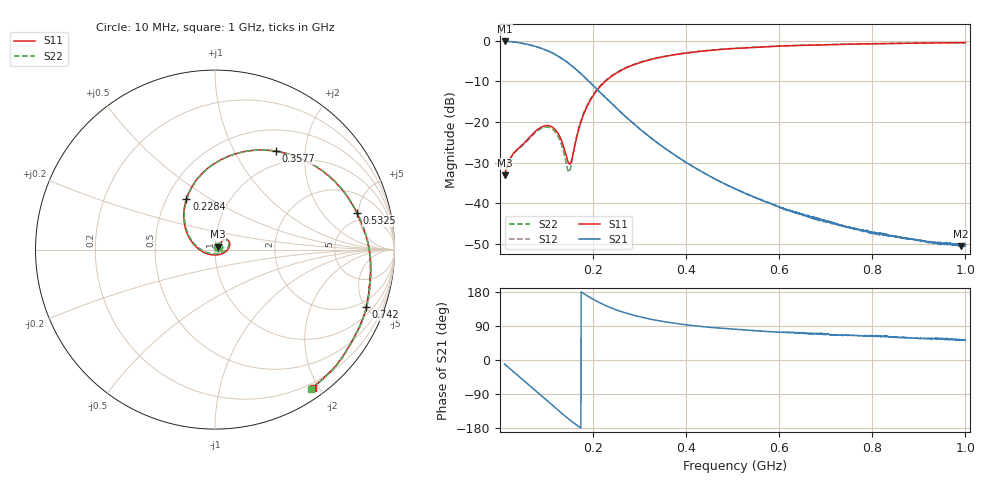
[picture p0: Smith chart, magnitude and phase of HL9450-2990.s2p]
! 7/13/2020 7:41:01 AM
! H:\PRODUCTION_DATA\9450\10009\HL9450_10009_117MHZ_.S2P
! CHANNEL.1
! TR.MEASUREMENT
! CORRECTED.DATA
# GHZ S RI R 50.0
! FREQ.GHZ  S11RE  S11IM  S21RE  S21IM  S12RE  S12IM  S22RE  S22IM
!; PortSelection: Port_12
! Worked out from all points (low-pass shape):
!   2000 points, 10 MHz to 1 GHz, reference 50 ohm
!   highest |S21| = -0.14 dB at 10 MHz (marker M1); lowest = -50.5 dB at 990.6 MHz (marker M2)
!   |S21| within 3 dB of the highest: start of sweep to 114.1 MHz
!   lowest |S11| = -33.1 dB at 10 MHz (marker M3), VSWR 1.05, Z = 51.5 + j1.71 ohm
!   |S11| at or under -10 dB: start of sweep to 226.6 MHz
!   |S22| runs from -33.1 to -0.5 dB; largest |S21 - S12| = 0.019
!   S11 on the Smith chart (normalised r, x): 10 MHz: 1.03, +0.03; 228.4 MHz: 0.63, +0.39; 357.7 MHz: 0.79, +1.48; 532.5 MHz: 3.91, +4.78; 742 MHz: 1.46, -5.03; 1 GHz: 0.14, -1.92
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0.01  0.0147 0.0166  0.9664 -0.1849  0.985 -0.188  0.0148 0.0164
0.02485743  0.0258 0.0279  0.8651 -0.433  0.8656 -0.4329  0.0259 0.0274
0.04714357  0.0339 0.039  0.5967 -0.7109  0.597 -0.7109  0.0333 0.0379
0.07784892  0.0534 0.057  0.1111 -0.8352  0.1113 -0.8355  0.0512 0.0558
0.09963982  0.0767 0.0475  -0.2046 -0.7332  -0.2045 -0.7332  0.0727 0.047
0.1174687  0.08 0.017  -0.3866 -0.5602  -0.3868 -0.5602  0.0747 0.0183
0.1298499  0.063 -0.00845  -0.456 -0.4168  -0.4569 -0.4169  0.0572 -0.00546
0.1481741  0.00625 -0.0301  -0.4774 -0.2114  -0.4776 -0.2109  0.000741 -0.0243
0.1546123  -0.0198 -0.0288  -0.4652 -0.148  -0.4656 -0.148  -0.0249 -0.0219
0.1754127  -0.1049 0.0147  -0.3844 0.00703  -0.3842 0.00707  -0.1072 0.0241
0.1976988  -0.164 0.1149  -0.2753 0.0908  -0.2752 0.0908  -0.1626 0.1253
0.2284042  -0.1596 0.2808  -0.1554 0.1178  -0.1555 0.1175  -0.154 0.2902
0.2828814  0.0176 0.4916  -0.0491 0.0868  -0.0492 0.0868  0.0276 0.4966
0.3403302  0.2658 0.5545  -0.0131 0.0527  -0.013 0.0527  0.2764 0.5545
0.3576638  0.3372 0.5484  -0.00828 0.0453  -0.00833 0.0454  0.3473 0.5475
0.5052476  0.7507 0.2744  0.00232 0.0149  0.00233 0.0149  0.757 0.2677
0.5324862  0.791 0.2037  0.0025 0.0126  0.00257 0.0126  0.7956 0.1954
0.6701651  0.8665 -0.1498  0.00236 0.00643  0.00228 0.00624  0.8658 -0.1587
0.741976  0.8429 -0.3209  0.0021 0.0047  0.00218 0.00475  0.842 -0.3301
0.8350825  0.7635 -0.511  0.00194 0.00357  0.00191 0.00354  0.7597 -0.5202
0.9905903  0.5585 -0.7566  0.00178 0.00238  0.00186 0.00246  0.5507 -0.764
1  0.5434 -0.7693  0.00192 0.00245  0.00189 0.0024  0.5356 -0.7752
